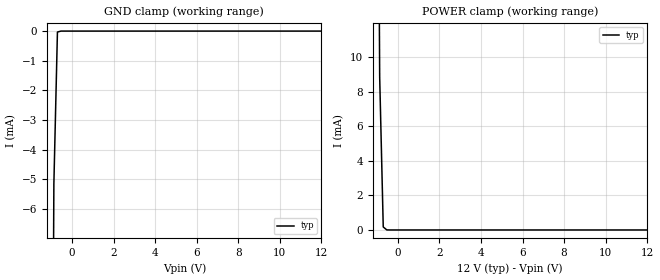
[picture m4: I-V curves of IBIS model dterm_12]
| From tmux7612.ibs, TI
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| dterm_12
[Model]   dterm_12
Model_type   Terminator
|   typ   min   max
C_comp   4.014581e-11   NA   NA
[Voltage Range]   12   NA   NA
[Temperature Range]   27   NA   NA
[Power Clamp Reference]   12   NA   NA
[GND Clamp Reference]   0   NA   NA
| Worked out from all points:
|   GND clamp passes 1 mA (typ) near -0.74 V on its own axis
|   POWER clamp passes 1 mA (typ) near -0.72 V on its own axis
[GND Clamp]
|   Voltage   I(typ)   I(min)   I(max)
-5V       -2.406A    NA         NA
-1.051V   -29.73mA   NA         NA
-878.8mV  -5.156mA   NA         NA
-707.1mV  -31.84uA   NA         NA
-535.4mV  -79.56nA   NA         NA
12V       108pA      NA         NA
[POWER Clamp]
|   Voltage   I(typ)   I(min)   I(max)
-5V       2.648A     NA         NA
-1.05V    45.5mA     NA         NA
-878.8mV  8.869mA    NA         NA
-707.1mV  174.1uA    NA         NA
-535.4mV  2.813uA    NA         NA
12V       -1.285nA   NA         NA
